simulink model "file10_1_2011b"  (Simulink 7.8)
settings: Solver=ode4  StartTime=0.0  StopTime=10  FixedStep=1e-3  RelTol=1e-3

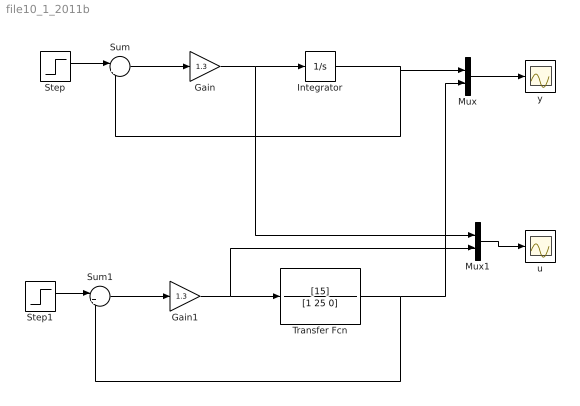
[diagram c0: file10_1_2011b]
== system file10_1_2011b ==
  Gain : Gain  Gain=1.3
  Gain1 : Gain  Gain=1.3
  Integrator : Integrator
  Mux : Mux  Inputs=2
  Mux1 : Mux  Inputs=2
  Step : Step  SampleTime=0
  Step1 : Step  SampleTime=0
  Sum : Sum  Inputs=|+-
  Sum1 : Sum  Inputs=|+-
  Transfer Fcn : TransferFcn  Numerator=[15]  Denominator=[1 25 0]
  u : Scope
  y : Scope
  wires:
  Integrator/1 -> Mux/1, Sum/2
  Transfer Fcn/1 -> Sum1/2, Mux/2
  Step1/1 -> Sum1/1
  Gain1/1 -> Transfer Fcn/1, Mux1/2
  Mux/1 -> y/1
  Mux1/1 -> u/1
  Step/1 -> Sum/1
  Sum/1 -> Gain/1
  Gain/1 -> Integrator/1, Mux1/1
  Sum1/1 -> Gain1/1
